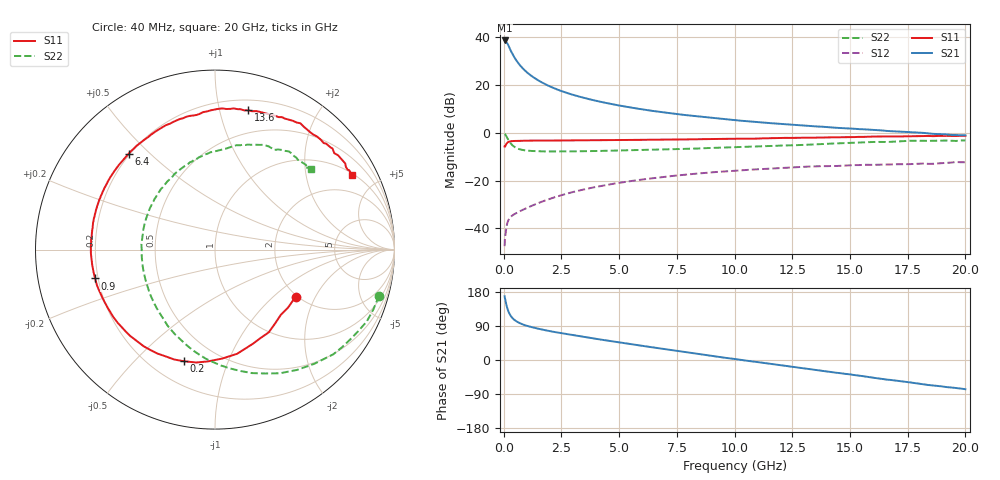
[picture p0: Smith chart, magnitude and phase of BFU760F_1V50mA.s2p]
! Filename:  P:\Prog\Test\Noise\ATS_data\Testdata_Net\Split files Spar\BFU760F_2W_C1_1V_5mA_60mA_Bias8_D.s2p
! Date/Time: Mon 06/Feb/2012 15:06:21
! BFU760_2W_C1_1V_5mA_60mA_Bias8_R.s2p
! MDIF S-parameter v. bias file
! BFU760_2W_C1_1V_5mA_60mA
! Date/time Fri Mar 18 10:56:44 2011
! VAR V_out= 1.0002
! VAR I_out= 49.9300
! VAR V_in= 0.8161
! VAR I_in= 0.1723
! Device data file deembeded for feedlines and parallel
! Original file: \Split files Spar\BFU760_2W_C1_1V_5mA_60mA_Bias8_R.s2p
! Feed-files: PR003V01_101208_Feed1.s2p, PR003V01_101208_Feed2.s2p
! Parallel-file: PR003V01_101208_Par.s2p
# MHz S MA R 50
!  Freq-MHz  S11-mag  S11-arg  S21-mag  S21-arg  S12-mag  S12-arg  S22-mag  S22-arg
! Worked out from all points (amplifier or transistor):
!   167 points, 40 MHz to 20 GHz, reference 50 ohm
!   highest |S21| = 38.7 dB at 40 MHz (marker M1)
!   |S21| within 3 dB of that: start of sweep to 245.1 MHz
!   unconditionally stable (mu >= 1): 2.951 GHz to 15.26 GHz
!   at 550 MHz: K = 0.49, MSG = 31.9 dB, |S12| = -33.5 dB
!   at 4.2 GHz: K = 1.03, MAG = 16.5 dB, |S12| = -22.2 dB
!   at 20 GHz: K = 0.96, MSG = 5.6 dB, |S12| = -12.3 dB
!   S11 on the Smith chart (normalised r, x): 40 MHz: 1.96, -1.41; 200 MHz: 0.33, -0.71; 900 MHz: 0.19, -0.11; 6.4 GHz: 0.20, +0.43; 13.6 GHz: 0.29, +1.23; 20 GHz: 1.06, +3.64
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40  0.52 -30.2  86.13 168.3  0.004259 79.8  0.9491 -15.7
50  0.5198 -38.4  84.21 163.9  0.005731 76.9  0.9433 -20.7
60  0.5163 -44.8  79.41 161.6  0.006302 73.3  0.9359 -25.2
80  0.5497 -57.1  82.79 155.7  0.007919 69.8  0.9048 -33.5
120  0.5934 -78.0  79.21 144.5  0.01085 62.2  0.8423 -49.2
160  0.6243 -93.7  73.76 135.8  0.0131 56.2  0.7783 -62.3
200  0.6455 -105.5  67.9 128.8  0.01474 51.7  0.7183 -73.3
260  0.6622 -119.0  58.85 120.9  0.0165 47.2  0.646 -87.2
300  0.6693 -126.3  53.33 116.8  0.01739 45.3  0.6094 -94.9
440  0.6784 -143.0  39.84 107.1  0.01965 42.1  0.5213 -115.5
600  0.681 -154.3  30.3 100.3  0.02168 42.5  0.4698 -130.9
900  0.6866 -166.5  20.68 92.3  0.02545 45.3  0.4322 -148.8
1250  0.6902 -175.0  15.02 86.1  0.03032 48.3  0.418 -161.2
1800  0.6921 176.0  10.47 78.6  0.03861 51.0  0.4102 -173.5
3400  0.7001 158.6  5.54 61.8  0.06432 49.3  0.4143 165.1
6400  0.7186 132.1  2.912 33.8  0.1118 34.3  0.4438 136.7
6800  0.7221 128.8  2.742 30.2  0.1179 31.7  0.449 133.3
10200  0.7576 102.0  1.814 0.9  0.1638 9.6  0.5061 106.0
13400  0.7927 78.2  1.381 -25.2  0.1987 -12.7  0.5721 82.5
13600  0.7979 76.5  1.361 -26.9  0.1993 -14.0  0.579 81.2
16800  0.8434 52.7  1.085 -52.9  0.2187 -34.9  0.6518 58.6
20000  0.8703 28.6  0.8903 -77.2  0.243 -56.3  0.6981 40.3
